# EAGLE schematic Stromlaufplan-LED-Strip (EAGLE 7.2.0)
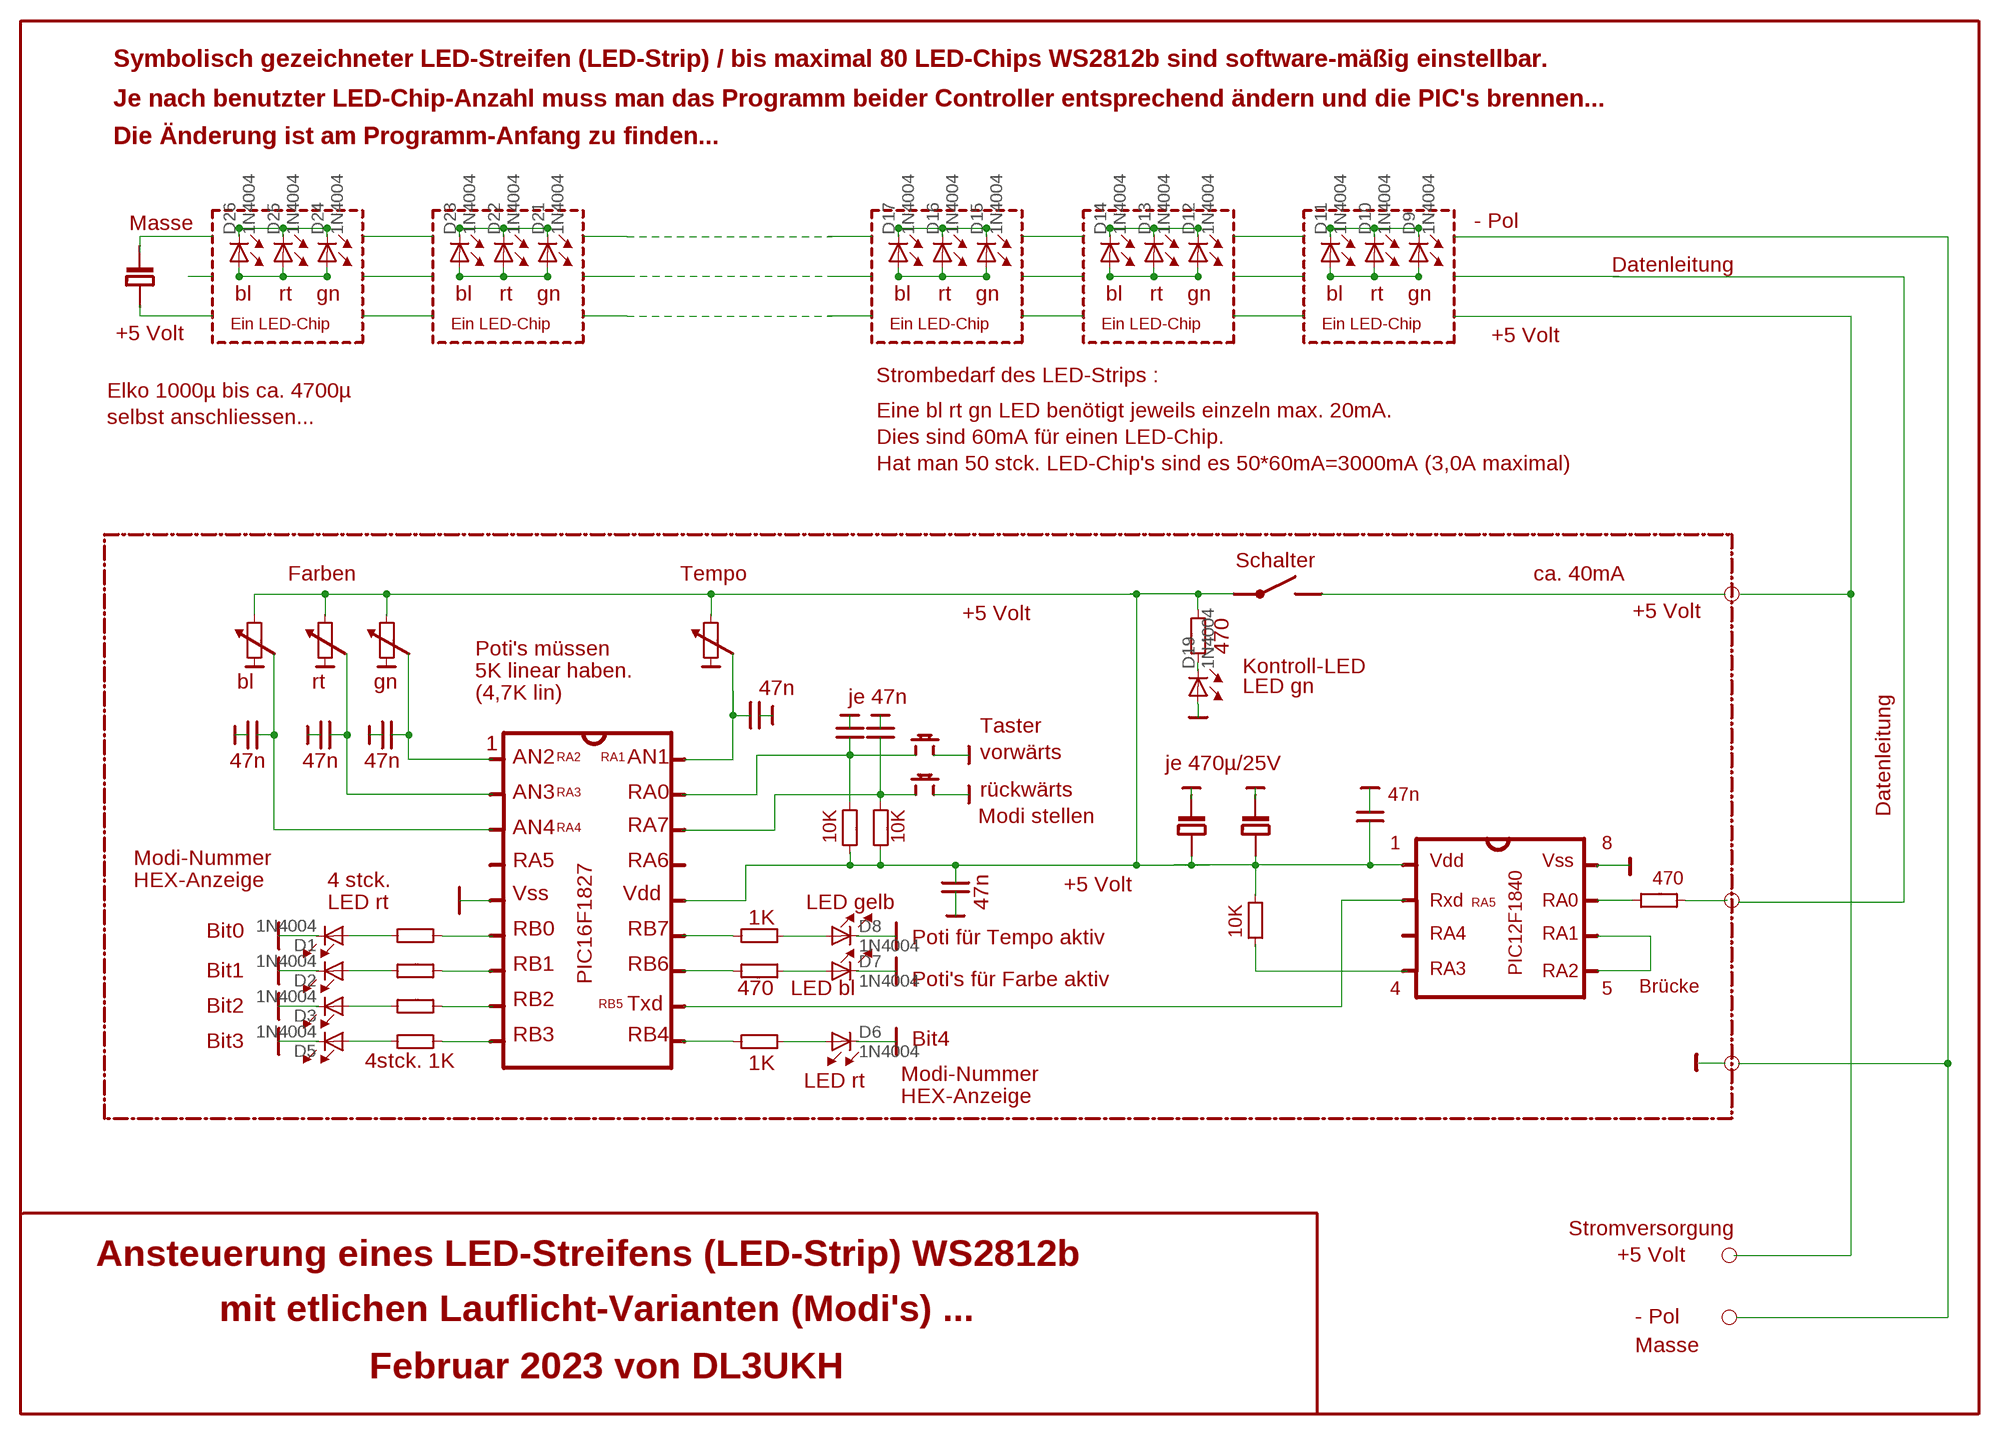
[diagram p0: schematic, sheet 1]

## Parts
D1  1N4004  [DO41-10]
D2  1N4004  [DO41-10]
D3  1N4004  [DO41-10]
D5  1N4004  [DO41-10]
D6  1N4004  [DO41-10]
D7  1N4004  [DO41-10]
D8  1N4004  [DO41-10]
D9  1N4004  [DO41-10]
D10  1N4004  [DO41-10]
D11  1N4004  [DO41-10]
D12  1N4004  [DO41-10]
D13  1N4004  [DO41-10]
D14  1N4004  [DO41-10]
D15  1N4004  [DO41-10]
D16  1N4004  [DO41-10]
D17  1N4004  [DO41-10]
D19  1N4004  [DO41-10]
D21  1N4004  [DO41-10]
D22  1N4004  [DO41-10]
D23  1N4004  [DO41-10]
D24  1N4004  [DO41-10]
D25  1N4004  [DO41-10]
D26  1N4004  [DO41-10]

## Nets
N$2: D1.A
N$3: D1.C
N$8: D2.A
N$9: D2.C
N$11: D3.A
N$12: D3.C
N$14: D5.A
N$15: D5.C
N$17: D6.A
N$18: D6.C
N$20: D7.A
N$21: D7.C
N$23: D8.A
N$24: D8.C
N$47: D9.A D10.A D11.A
N$48: D12.A D13.A D14.A
N$49: D12.C D13.C D14.C
N$50: D9.C D10.C D11.C
N$52: D15.A D16.A D17.A
N$53: D15.C D16.C D17.C
N$58: D21.A D22.A D23.A
N$59: D21.C D22.C D23.C
N$61: D24.A D25.A D26.A
N$62: D24.C D25.C D26.C
N$69: D19.C
N$72: D19.A

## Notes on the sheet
- Symbolisch gezeichneter LED-Streifen (LED-Strip) / bis maximal 80 LED-Chips WS2812b sind software-mäßig einstellbar.
- Je nach benutzter LED-Chip-Anzahl muss man das Programm beider Controller entsprechend ändern und die PIC's brennen...
- Die Änderung ist am Programm-Anfang zu finden...
- Masse | - Pol
- Datenleitung
- bl | rt | gn | bl | rt | gn | bl | rt | gn | bl | rt | gn | bl | rt | gn
- Ein LED-Chip | Ein LED-Chip | Ein LED-Chip | Ein LED-Chip | Ein LED-Chip | +5 Volt
- +5 Volt
- Strombedarf des LED-Strips :
- Elko 1000µ bis ca. 4700µ
- Eine bl rt gn LED benötigt jeweils einzeln max. 20mA.
- selbst anschliessen...
- Dies sind 60mA für einen LED-Chip.
- Hat man 50 stck. LED-Chip's sind es 50*60mA=3000mA (3,0A maximal)
- Schalter
- Farben | Tempo | ca. 40mA
- +5 Volt | 470 | +5 Volt
- Poti's müssen
- 5K linear haben. | Kontroll-LED
- 47n
- bl | rt | gn | je 47n | LED gn
- (4,7K lin)
- Taster
- 47n | 47n | 47n | 1
- AN2 | RA2 | RA1 | AN1 | vorwärts
- je 470µ/25V
- AN3 | RA3 | RA0 | rückwärts
- 47n
- Datenleitung
- Modi stellen
- AN4 | RA4 | RA7
- 10K | 10K
- 1 | 8
- Modi-Nummer | RA5 | RA6 | Vdd | Vss
- 47n
- HEX-Anzeige | 4 stck. | 470
- +5 Volt
- Vss | Vdd | RA5
- LED rt | LED gelb | Rxd | RA0
- 1K
- Bit0 | RB0 | RB7 | 10K | RA4 | RA1
- Poti für Tempo aktiv
- RB1 | RB6 | RA3 | PIC12F1840
- Bit1 | RA2
- PIC16F1827 | Poti's für Farbe aktiv
- 470 | LED bl | 4 | 5 | Brücke
- RB2 | RB5 | Txd
- Bit2
- RB3 | RB4 | Bit4
- Bit3
- 4stck. 1K | 1K
- Modi-Nummer
- LED rt
- HEX-Anzeige
- Stromversorgung
- Ansteuerung eines LED-Streifens (LED-Strip) WS2812b | +5 Volt
- mit etlichen Lauflicht-Varianten (Modi's) ... | - Pol
- Masse
- Februar 2023 von DL3UKH

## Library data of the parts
D1-D3 D5-D17 D19 D21-D26 = diode:1N4004: DIODE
